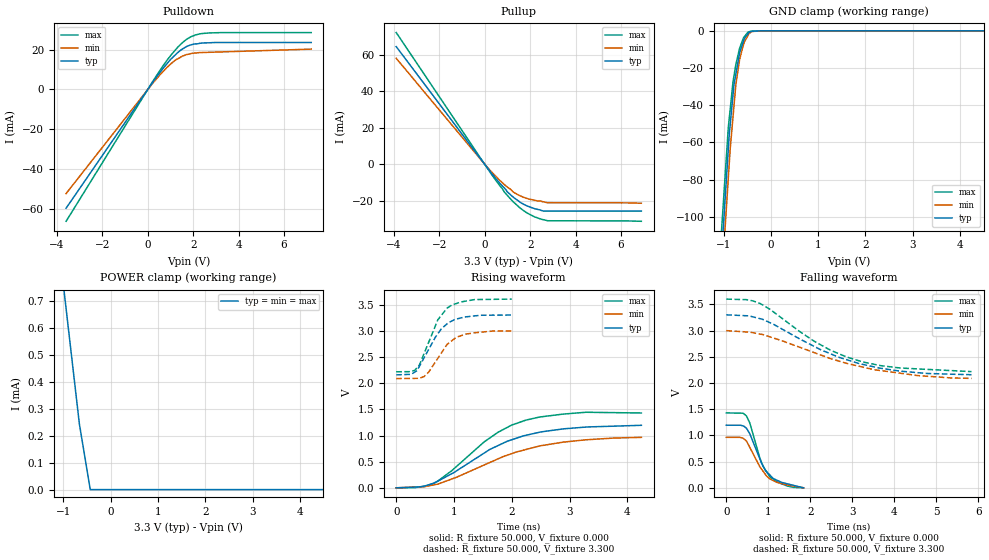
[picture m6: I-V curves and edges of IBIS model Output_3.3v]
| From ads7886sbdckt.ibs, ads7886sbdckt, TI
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[Model] Output_3.3v
Model_type 3-state
Vref=0.00000V
Rref=5.00000Mohms
Cref=50.0000pF
Vmeas=1.65000V
C_comp 1.513pF 1.513pF 1.513pF
| variable typ   min   max
[Voltage Range] 3.30000V 3.00000V 3.60000V
[POWER Clamp Reference] 3.30000V 3.00000V 3.60000V
[Pullup Reference] 3.30000V 3.00000V 3.60000V
[Pulldown Reference] 0.00000V 0.00000V 0.00000V
[GND Clamp Reference] 0.00000V 0.00000V 0.00000V
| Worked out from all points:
|   slope of the pulldown table from 0 to 0.495 V, typ, clamps not added: 62.9 ohm
|   slope of the pullup table from 0 to 0.495 V, typ, clamps not added: 62.9 ohm
|   GND clamp passes 1 mA (typ) near -0.47 V on its own axis
|   rising waveform, R_fixture 50.000, V_fixture 0.000: 20-80 % time 1.19ns typ, 1.36ns min, 993ps max; typ from 0 V to 1.2 V
|   falling waveform, R_fixture 50.000, V_fixture 0.000: 20-80 % time 446ps typ, 445ps min, 383ps max; typ from 1.2 V to 0 V
|   falling waveform, R_fixture 50.000, V_fixture 3.300: 20-80 % time 1.87ns typ, 2.15ns min, 1.7ns max; typ from 3.3 V to 2.16 V
|   rising waveform, R_fixture 50.000, V_fixture 3.300: 20-80 % time 383ps typ, 372ps min, 348ps max; typ from 2.16 V to 3.3 V
[GND Clamp]
-3.6V     -1.139A    -1.146A    -1.1A
-3V       -900.1mA   -909.1mA   -867.3mA
-900mV    -64.03mA   -79.55mA   -52.21mA
-860mV    -50.67mA   -63.75mA   -42.33mA
-800mV    -34.5mA    -46.36mA   -27.5mA
-780mV    -29.11mA   -40.56mA   -24.4mA
-740mV    -23.33mA   -28.97mA   -18.18mA
-660mV    -11.76mA   -15.42mA   -9.404mA
-560mV    -4.133mA   -6.021mA   -3.198mA
-480mV    -1.448mA   -2.358mA   -610uA
-200mV    0A         0A         0A
7.2V      0A         0A         0A
[Pulldown]
-3.6V     -59.6mA    -52.25mA   -66.17mA
200mV     3.304mA    2.851mA    3.682mA
580mV     9.182mA    7.879mA    10.29mA
1V        15.01mA    12.68mA    16.86mA
1.26V     17.83mA    15.06mA    20.38mA
1.44V     19.61mA    16.14mA    22.51mA
1.7V      21.44mA    17.43mA    25.05mA
2.08V     22.85mA    18.23mA    27.26mA
2.72V     23.38mA    18.62mA    28.33mA
7.2V      23.53mA    20.21mA    28.51mA
[Pullup]
|  Voltage   I(typ)   I(min)   I(max)
-3.9V     64.5mA     58.1mA     72.2mA
300mV     -4.95mA    -4.14mA    -5.52mA
980mV     -14.9mA    -12.3mA    -16.8mA
1.26V     -18mA      -15.2mA    -20.6mA
1.66V     -21.5mA    -17.8mA    -24.9mA
2.2V      -24.3mA    -19.7mA    -28.8mA
2.58V     -25.6mA    -20.5mA    -30.3mA
2.76V     -25.6mA    -21mA      -30.9mA
6.9V      -25.6mA    -21.3mA    -31.2mA
[POWER Clamp]
-3.9V     5.179mA    5.179mA    5.179mA
-2.7V     3.351mA    3.351mA    3.351mA
-860mV    548.4uA    548.4uA    548.4uA
-660mV    243.7uA    243.7uA    243.7uA
-430mV    0A         0A         0A
6.9V      0A         0A         0A
[Rising Waveform]
R_fixture = 50.000
V_fixture = 0.000
V_fixture_min = 0.000
V_fixture_max = 0.000
|  time   V(typ)   V(min)   V(max)
0s        189uV      1.42mV     -151.4uV
480ps     33.21mV    19.81mV    23.81mV
640ps     85.71mV    54.38mV    82.5mV
960ps     270.4mV    168.6mV    327.2mV
1.52ns    663.4mV    436mV      877.2mV
1.76ns    807.1mV    553.6mV    1.061V
2.24ns    1.003V     731.4mV    1.293V
2.88ns    1.125V     872.3mV    1.408V
3.28ns    1.161V     917.9mV    1.444V
4.24ns    1.195V     964.3mV    1.43V
[Falling Waveform]
R_fixture = 50.000
V_fixture = 0.000
V_fixture_min = 0.000
V_fixture_max = 0.000
|  time   V(typ)   V(min)   V(max)
0s        1.195V     964.3mV    1.43V
320ps     1.195V     964.3mV    1.425V
480ps     1.136V     892.5mV    1.372V
560ps     1.031V     769.6mV    1.236V
800ps     550.5mV    400.9mV    563.6mV
940ps     323.5mV    245.6mV    329.8mV
1.04ns    242.2mV    169.2mV    208.3mV
1.12ns    177.2mV    137.7mV    161.4mV
1.44ns    79.63mV    56.61mV    37.96mV
1.84ns    189uV      1.42mV     -151.4uV
[Falling Waveform]
R_fixture = 50.000
V_fixture = 3.300
V_fixture_min = 3.000
V_fixture_max = 3.600
|  time   V(typ)   V(min)   V(max)
0s        3.3V       2.999V     3.6V
480ps     3.283V     2.974V     3.59V
800ps     3.228V     2.934V     3.519V
1.14ns    3.113V     2.854V     3.346V
2.08ns    2.704V     2.584V     2.803V
2.48ns    2.558V     2.466V     2.626V
3.16ns    2.371V     2.32V      2.424V
4.14ns    2.226V     2.187V     2.286V
4.56ns    2.197V     2.141V     2.269V
5.84ns    2.158V     2.088V     2.217V
[Rising Waveform]
R_fixture = 50.000
V_fixture = 3.300
V_fixture_min = 3.000
V_fixture_max = 3.600
|  time   V(typ)   V(min)   V(max)
0s        2.158V     2.088V     2.217V
260ps     2.169V     2.091V     2.226V
360ps     2.239V     2.092V     2.294V
400ps     2.32V      2.092V     2.343V
560ps     2.641V     2.208V     2.776V
720ps     2.944V     2.475V     3.21V
880ps     3.134V     2.741V     3.434V
960ps     3.186V     2.809V     3.491V
1.2ns     3.266V     2.936V     3.566V
2ns       3.301V     2.999V     3.605V
[Ramp]
| variable typ min max
dV/dt_r 716.796m/958.384p 576.718m/1.10016n 858.231m/871.807p
dV/dt_f 685.293m/1.82567n 546.383m/2.13248n 829.523m/1.58806n
R_load = 50.0000Ohms
